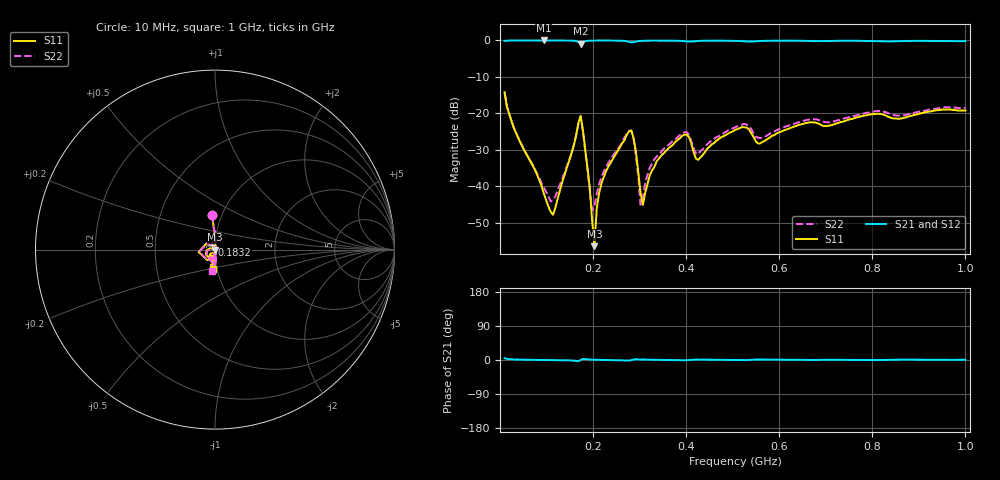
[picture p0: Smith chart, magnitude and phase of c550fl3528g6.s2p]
!Agilent Technologies,N5234A,MY52241123,A.10.00.00
!Agilent N5234A: A.10.00.00
!Date: Friday, January 04, 2019 08:09:03
!Correction: S11(Full 2 Port(1,2))
!S21(Full 2 Port(1,2))
!S12(Full 2 Port(1,2))
!S22(Full 2 Port(1,2))
!S2P File: Measurements: S11, S21, S12, S22:
# Hz S  dB  R 50
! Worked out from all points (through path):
!   201 points, 10 MHz to 1 GHz, reference 50 ohm
!   highest |S21| = -0.01 dB at 94.15 MHz (marker M1); lowest = -0.9 dB at 173.3 MHz (marker M2)
!   lowest |S11| = -56.5 dB at 203.1 MHz (marker M3), VSWR 1.00, Z = 50.1 - j0.106 ohm
!   |S11| at or under -10 dB: start of sweep to end of sweep
!   |S22| runs from -46.6 to -14.4 dB; largest |S21 - S12| = 0.0031
!   S11 on the Smith chart (normalised r, x): 10 MHz: 0.90, +0.36; 183.2 MHz: 0.96, +0.05; 1 GHz: 0.95, -0.21
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1e7  -14.24 94.8  -0.13 4.6  -0.12 4.7  -14.37 94.7
9.415e7  -41.98 66.8  -0.01 0.1  -0.01 0.1  -40.34 54.1
1.1395e8  -47.85 -7.4  -0.01 -0.1  -0.01 -0.2  -43.84 -6.4
1.7335e8  -20.70 -171.6  -0.89 -0.2  -0.89 -0.2  -20.98 -171.9
1.783e8  -24.63 143.5  -0.46 2.7  -0.46 2.7  -25.02 140.7
1.8325e8  -29.98 123.6  -0.20 2.2  -0.20 2.2  -30.48 117.2
1.981e8  -49.56 93.1  -0.05 0.9  -0.05 0.9  -46.63 37.4
2.0305e8  -56.47 -44.9  -0.04 0.7  -0.04 0.7  -45.54 -16.9
2.08e8  -46.04 -68.1  -0.04 0.6  -0.04 0.5  -42.09 -39.6
2.179e8  -39.34 -76.0  -0.03 0.3  -0.03 0.3  -37.58 -58.1
2.773e8  -24.96 -128.8  -0.38 -1.4  -0.37 -1.4  -24.74 -121.1
2.872e8  -26.81 -177.4  -0.48 1.2  -0.48 1.2  -27.21 -170.2
3.0205e8  -41.82 177.4  -0.14 1.5  -0.14 1.5  -45.07 -149.7
3.07e8  -45.16 -143.2  -0.10 1.3  -0.10 1.2  -43.20 -92.6
3.4165e8  -32.43 -86.7  -0.04 0.4  -0.04 0.4  -31.28 -74.3
4.0105e8  -25.82 -118.8  -0.27 -0.5  -0.27 -0.5  -25.14 -108.0
4.258e8  -32.79 -111.4  -0.14 1.1  -0.15 1.1  -31.22 -101.4
5.05e8  -24.58 -94.7  -0.10 -0.3  -0.11 -0.3  -23.85 -88.7
5.5945e8  -28.27 -105.6  -0.16 1.2  -0.16 1.2  -26.77 -100.3
6.733e8  -22.50 -100.0  -0.17 0.0  -0.18 0.0  -21.60 -95.6
8.3665e8  -21.07 -104.6  -0.27 0.6  -0.28 0.6  -20.10 -103.2
1e9  -19.24 -96.0  -0.19 0.7  -0.19 0.7  -18.54 -97.1
